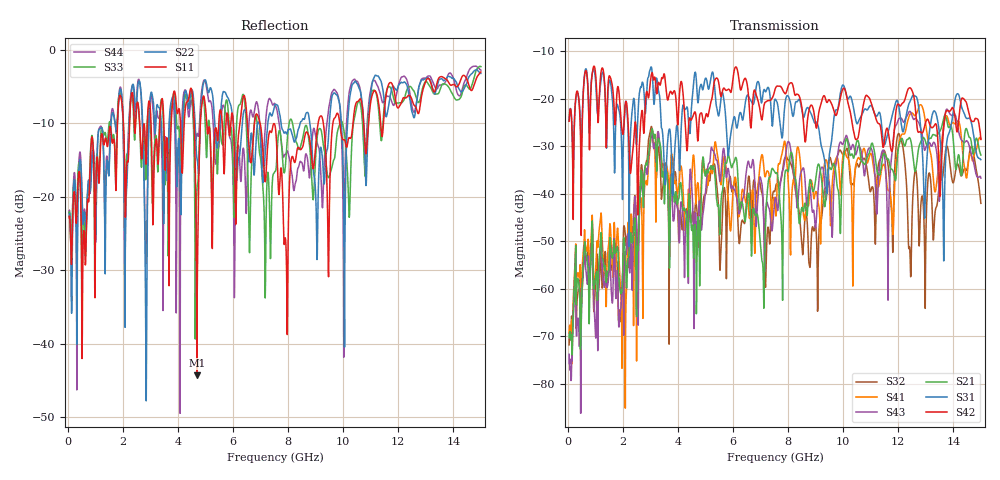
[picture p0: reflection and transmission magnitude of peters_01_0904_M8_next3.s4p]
# MHZ S RI R 50.00
! FREQ  S11  S12  S13  S14
!  S21  S22  S23  S24
!  S31  S32  S33  S34
!  S41  S42  S43  S44
!  REAL  IMAG  REAL  IMAG  REAL  IMAG  REAL  IMAG
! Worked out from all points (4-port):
!   1496 points, 50 MHz to 15 GHz, reference 50 ohm
!   strongest paths, dB at 50 MHz, 3.79 GHz, 7.53 GHz, 11.27 GHz, 15 GHz:
!     S42: -24.7, -19.0, -17.9, -25.1, -28.5
!     S31: -24.6, -37.0, -20.1, -23.1, -32.8
!     S21: -70.4, -36.3, -35.5, -35.8, -31.8
!     S43: -73.8, -39.7, -40.9, -38.3, -36.7
!     S41: -69.4, -31.9, -42.3, -38.6, -28.4
!     S32: -71.8, -32.8, -39.2, -34.2, -42.0
!   lowest |S11| = -44.3 dB at 4.69 GHz (marker M1), VSWR 1.01, Z = 49.4 + j0.101 ohm
!   |S11| at or under -10 dB: start of sweep to 1.806 GHz; 6.981 GHz to 9.092 GHz (2.111 GHz wide, 26.3 % of centre); 9.876 GHz to 10.36 GHz (481.3 MHz wide, 4.76 % of centre)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
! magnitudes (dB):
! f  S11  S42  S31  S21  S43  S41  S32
! 50 MHz  -22.9  -24.7  -24.6  -70.4  -73.8  -69.4  -71.8
! 2.03 GHz  -10.7  -26.5  -26.9  -49.3  -69.9  -52.4  -47.1
! 2.61 GHz  -9.9  -28.7  -18.5  -42.1  -42.5  -43.4  -40.0
! 2.84 GHz  -15.6  -19.4  -21.4  -33.7  -34.6  -37.3  -33.5
! 3.08 GHz  -21.3  -14.7  -15.6  -26.6  -28.0  -26.8  -27.4
! 4.69 GHz  -44.3  -26.1  -17.9  -54.3  -51.9  -38.6  -43.5
! 15 GHz  -3.0  -28.5  -32.8  -31.8  -36.7  -28.4  -42.0
